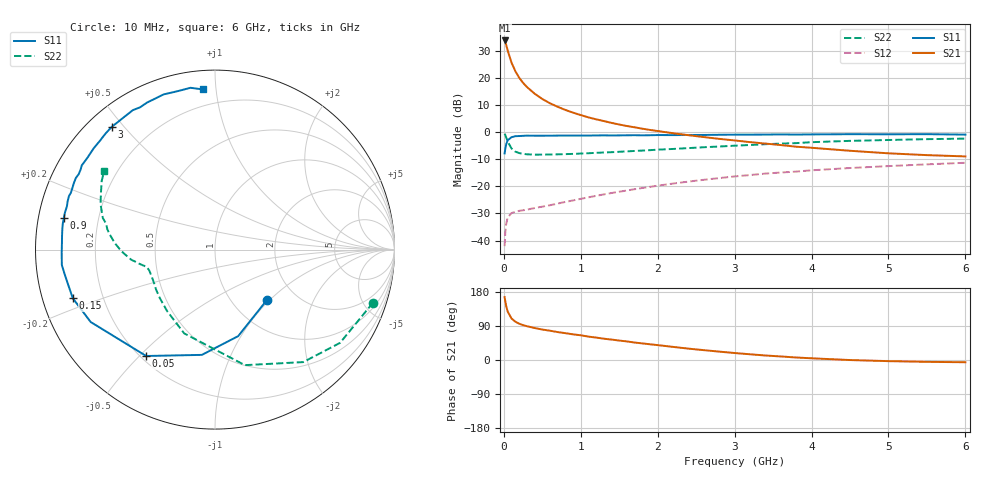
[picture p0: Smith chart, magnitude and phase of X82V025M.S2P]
! SIEMENS Small Signal Semiconductors
! BFP136W
! Si NPN RF Bipolar Junction Transistor in SOT343
! VCE = 2 V  IC = 25 mA
! Common Emitter S-Parameters:  September  1994
# GHz  S  MA  R  50
!  f  S11  S21  S12  S22
! GHz  MAG  ANG  MAG  ANG  MAG  ANG  MAG  ANG
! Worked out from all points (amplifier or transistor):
!   40 points, 10 MHz to 6 GHz, reference 50 ohm
!   highest |S21| = 33.7 dB at 10 MHz (marker M1)
!   |S21| within 3 dB of that: start of sweep to 43.42 MHz
!   unconditionally stable (mu >= 1): 777.5 MHz to 2.779 GHz
!   at 200 MHz: K = 0.39, MSG = 24.5 dB, |S12| = -29.0 dB
!   at 1.5 GHz: K = 1.16, MAG = 10.0 dB, |S12| = -22.0 dB
!   at 6 GHz: K = 0.99, MSG = 1.2 dB, |S12| = -11.3 dB
!   S11 on the Smith chart (normalised r, x): 10 MHz: 1.44, -0.96; 50 MHz: 0.22, -0.52; 150 MHz: 0.09, -0.17; 900 MHz: 0.08, +0.10; 3 GHz: 0.07, +0.46; 6 GHz: 0.10, +0.92
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0.01  0.4031 -44.0  48.46 166.1  0.0079 74.4  0.9285 -18.6
0.02  0.4991 -75.0  44.37 153.4  0.0149 64.6  0.8692 -36.7
0.03  0.5911 -97.1  40.4 142.9  0.02 55.9  0.7965 -51.9
0.05  0.706 -122.9  31.66 127.7  0.0266 42.3  0.6649 -75.5
0.1  0.8017 -149.8  18.91 109.5  0.0322 29.3  0.4973 -110.2
0.15  0.8373 -161.1  13.14 101.0  0.0338 26.7  0.4338 -128.1
0.2  0.8419 -167.1  9.939 95.7  0.0353 25.8  0.4089 -138.9
0.25  0.8501 -171.3  8.038 92.0  0.0362 26.4  0.3966 -145.9
0.3  0.8577 -174.3  6.737 89.2  0.0371 27.8  0.3882 -150.6
0.4  0.8542 -179.1  5.076 84.4  0.0398 31.2  0.3833 -156.6
0.5  0.8536 177.4  4.049 80.4  0.0422 34.6  0.3834 -160.4
0.6  0.8555 175.0  3.379 77.3  0.0448 37.5  0.3845 -162.5
0.7  0.8584 172.2  2.91 73.7  0.0481 40.6  0.3876 -163.9
0.9  0.8603 168.1  2.272 67.7  0.0549 44.7  0.3954 -166.2
1.1  0.8596 163.7  1.856 61.7  0.0627 48.5  0.4065 -167.3
1.5  0.8656 156.7  1.373 51.3  0.0794 52.3  0.432 -169.7
2.2  0.8758 144.2  0.949 34.6  0.1123 52.8  0.4872 -175.2
3  0.8936 130.1  0.699 18.4  0.1519 48.3  0.5596 176.3
3.2  0.8936 126.8  0.651 15.1  0.1612 46.7  0.5762 173.9
4.5  0.9108 108.3  0.451 -0.1  0.2171 35.2  0.6864 158.3
5.5  0.9118 98.6  0.375 -4.9  0.2536 26.9  0.7382 148.8
6  0.895 94.4  0.355 -5.9  0.2711 22.3  0.756 144.8
